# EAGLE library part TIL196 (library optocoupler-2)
TEXAS INSTRUMENTS OPTO COUPLER
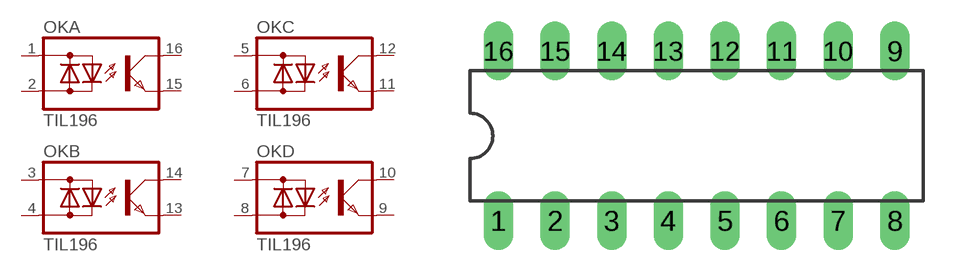
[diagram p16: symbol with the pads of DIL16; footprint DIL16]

Designator prefix OK; gates A=OK-LD B=OK-LD C=OK-LD D=OK-LD

## TIL196  [DIL16]
1  A:AC1  pas
2  A:AC2  pas
3  B:AC1  pas
4  B:AC2  pas
5  C:AC1  pas
6  C:AC2  pas
7  D:AC1  pas
8  D:AC2  pas
9  D:E  pas
10  D:C  pas
11  C:E  pas
12  C:C  pas
13  B:E  pas
14  B:C  pas
15  A:E  pas
16  A:C  pas

## Footprint DIL16 (pad centres in mm)
Dual In Line Package
drill 0.813 long: 1 -8.89,-3.81; 2 -6.35,-3.81; 3 -3.81,-3.81; 4 -1.27,-3.81; 5 1.27,-3.81; 6 3.81,-3.81; 7 6.35,-3.81; 8 8.89,-3.81; 9 8.89,3.81; 10 6.35,3.81; 11 3.81,3.81; 12 1.27,3.81; 13 -1.27,3.81; 14 -3.81,3.81; 15 -6.35,3.81; 16 -8.89,3.81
